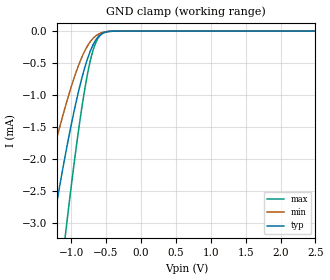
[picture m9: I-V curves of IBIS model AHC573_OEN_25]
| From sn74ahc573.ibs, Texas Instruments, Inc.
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[Model]   AHC573_OEN_25
Model_type  Input
Vinl=0.7
Vinh=1.7
| variable   typ   min   max
C_comp   0.75pF   0.68pF   0.81pF
[Temperature Range]   40   100   -40
| Ambient temperature   25   85   -40
[Voltage range]   2.5   2.3   2.7
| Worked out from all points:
|   GND clamp passes 1 mA (typ) near -0.91 V on its own axis
[GND Clamp]
| AHC573_OEN_25
|   Voltage   I(typ)   I(min)   I(max)
-2.5V     -13.29mA   -8.66mA    -18.97mA
-1.525V   -4.9mA     -3.136mA   -7.711mA
-1.285V   -3.194mA   -2.012mA   -5.171mA
-1.255V   -2.995mA   -1.881mA   -4.865mA
-1.085V   -1.941mA   -1.184mA   -3.204mA
-1.06V    -1.798mA   -1.09mA    -2.971mA
-940mV    -1.159mA   -673.8uA   -1.916mA
-805mV    -569.6uA   -310.1uA   -907.1uA
-710mV    -270.8uA   -143.8uA   -393uA
-610mV    -85.86uA   -49.23uA   -103.2uA
-415mV    -3.024uA   -2.096uA   -1.885uA
2.5V      1.669nA    486pA      4.202nA
